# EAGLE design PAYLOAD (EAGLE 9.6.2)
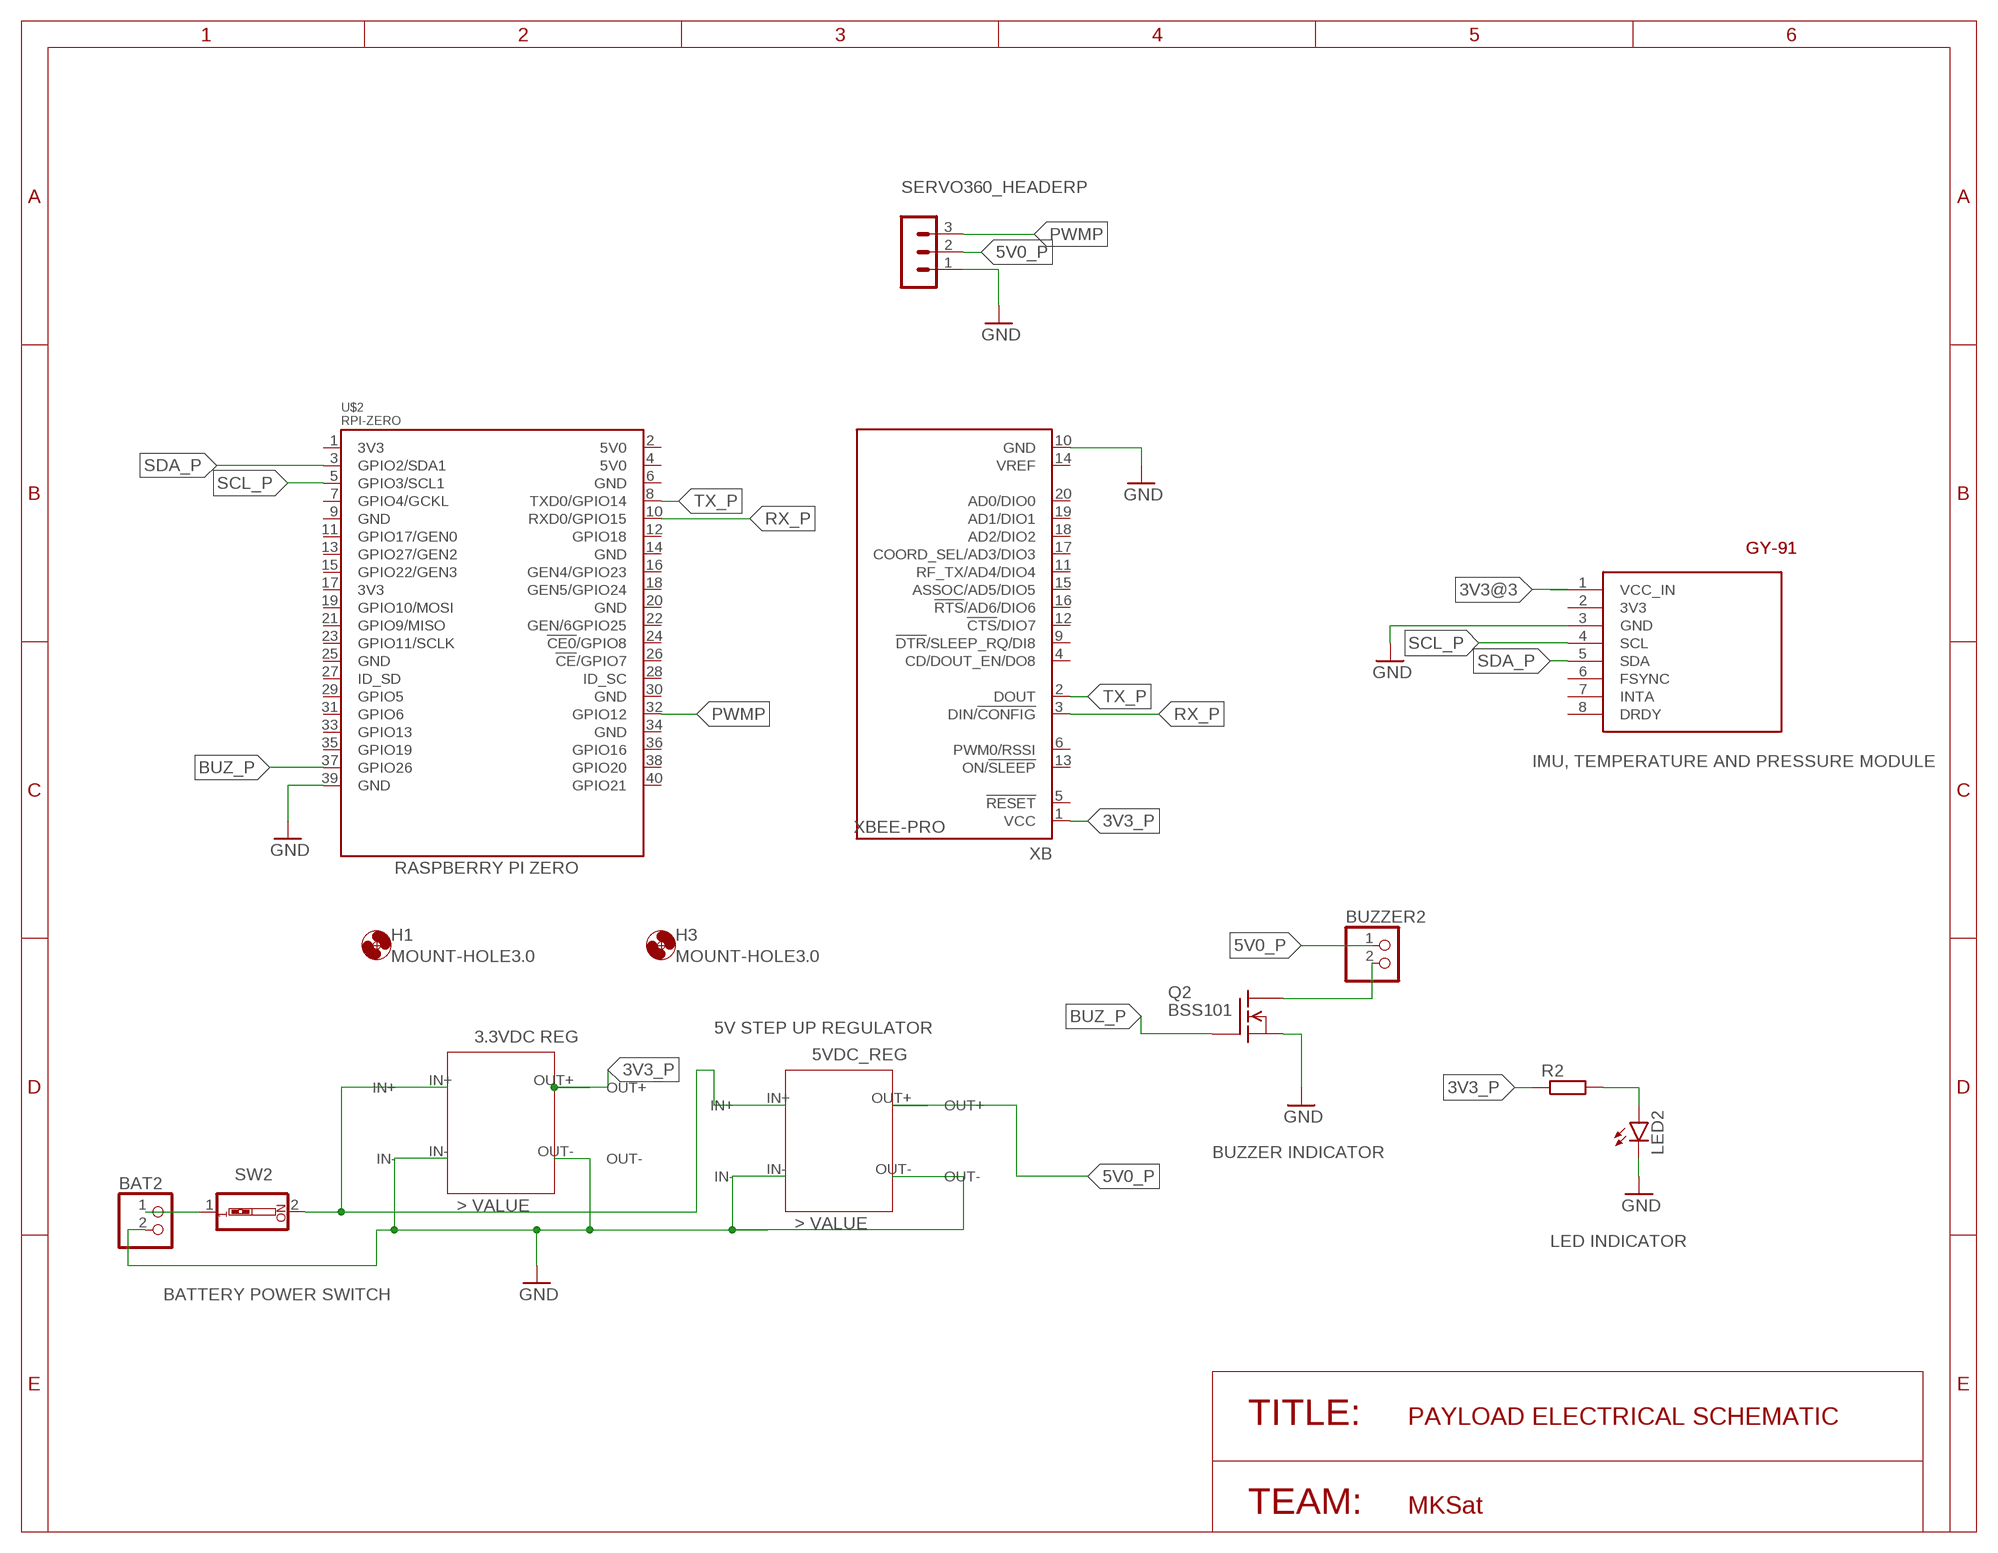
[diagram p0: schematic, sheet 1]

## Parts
BAT2  PINHD-1X2/90  [1X02/90]
BUZZER2  PINHD-1X2/90  [1X02/90]
GY-91  GY-86  [GY-86]
H1  MOUNT-HOLE3.0  [3,0]
H3  MOUNT-HOLE3.0  [3,0]
LED2  LED5MM  [LED5MM]
Q2  BSS101  [TO92]
R2  R-EU_0207/12  [0207/12]
SERVO360_HEADERP  MA03-1  [MA03-1]
SW2  SW_DIP-1  [EDG-01]
U$1  3VDC_REG  [3VDC_REG]
U$2  RPI-ZERO  [RASPBERRYPI_BASTELSTUBE_V13_RASPI_BOARD_B+_FULL]
U$3  5VDC_REG  [5VDC_REG]
XB  XBEE-PRO  [XBEE-PRO]

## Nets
3V3@3: GY-91.1(VCC_IN)
3V3_P: R2.1 U$1.OUT+ XB.1(VCC)
5V0_P: BUZZER2.1 SERVO360_HEADERP.2 U$3.OUT+
BUZ_P: Q2.2(G) U$2.37(GPIO26)
GND: BAT2.2 GY-91.3(GND) LED2.K(C) Q2.1(S) SERVO360_HEADERP.1 U$1.IN- U$1.OUT- U$2.39(GND) U$3.IN- U$3.OUT- XB.10(GND)
N$1: BUZZER2.2 Q2.3(D)
N$2: SW2.2 U$1.IN+ U$3.IN+
N$3: BAT2.1 SW2.1
N$11: LED2.A R2.2
PWMP: SERVO360_HEADERP.3 U$2.32(GPIO12)
RX_P: U$2.10(RXD0/GPIO15) XB.3(DIN/!CONFIG)
SCL_P: GY-91.4(SCL) U$2.5(GPIO3/SCL1)
SDA_P: GY-91.5(SDA) U$2.3(GPIO2/SDA1)
TX_P: U$2.8(TXD0/GPIO14) XB.2(DOUT)
Unconnected: GY-91.2(3V3) GY-91.6(FSYNC) GY-91.7(INTA) GY-91.8(DRDY) U$2.1(3V3) U$2.2(5V0) U$2.4(5V0) U$2.6(GND) U$2.7(GPIO4/GCKL) U$2.9(GND) U$2.11(GPIO17/GEN0) U$2.12(GPIO18) U$2.13(GPIO27/GEN2) U$2.14(GND) U$2.15(GPIO22/GEN3) U$2.16(GEN4/GPIO23) U$2.17(3V3) U$2.18(GEN5/GPIO24) U$2.19(GPIO10/MOSI) U$2.20(GND) U$2.21(GPIO9/MISO) U$2.22(GEN/6GPIO25) U$2.23(GPIO11/SCLK) U$2.24(!CE0!/GPIO8) U$2.25(GND) U$2.26(!CE!/GPIO7) U$2.27(ID_SD) U$2.28(ID_SC) U$2.29(GPIO5) U$2.30(GND) U$2.31(GPIO6) U$2.33(GPIO13) U$2.34(GND) U$2.35(GPIO19) U$2.36(GPIO16) U$2.38(GPIO20) U$2.40(GPIO21) XB.4(CD/DOUT_EN/DO8) XB.5(!RESET) XB.6(PWM0/RSSI) XB.9(!DTR!/SLEEP_RQ/DI8) XB.11(RF_TX/AD4/DIO4) XB.12(!CTS!/DIO7) XB.13(ON/!SLEEP) XB.14(VREF) XB.15(ASSOC/AD5/DIO5) XB.16(!RTS!/AD6/DIO6) XB.17(COORD_SEL/AD3/DIO3) XB.18(AD2/DIO2) XB.19(AD1/DIO1) XB.20(AD0/DIO0)

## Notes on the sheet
- GY-91 | GY-91
- IMU, TEMPERATURE AND PRESSURE MODULE
- RASPBERRY PI ZERO
- 5V STEP UP REGULATOR
- BUZZER INDICATOR
- LED INDICATOR
- BATTERY POWER SWITCH
- TITLE: | PAYLOAD ELECTRICAL SCHEMATIC
- TEAM: | MKSat

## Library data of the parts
BAT2 BUZZER2 = pinhead:PINHD-1X2: PIN HEADER
GY-91 = GY_Boards:GY-86
H1 H3 = holes:MOUNT-HOLE: MOUNTING HOLE with drill center marker
LED2 = led:LED: LED
Q2 = transistor-fet:BSS101: N-Channel Enhancement MOSFET 200V; 0,16A; 11Ohm
R2 = rcl:R-EU_: RESISTOR, European symbol; SPICEPREFIX: R
SERVO360_HEADERP = con-lstb:MA03-1: PIN HEADER; OC_FARNELL: unknown; OC_NEWARK: unknown
SW2 = special:SW_DIP-1: DIP SWITCH
U$1 = VOLTAGE_REGULATORS_CANSAT:3VDC_REG
U$2 = RPI-Zero:RPI-ZERO
U$3 = VOLTAGE_REGULATORS_CANSAT:5VDC_REG
XB = maxstream:XBEE: XBee (TM) /XBee-PRO(TM) OEM RF Modules Source: MaxStream, Inc. xbee_productmanual.pdf; MPN: XBP24-AWI-001; OC_FARNELL: 1337916; OC_NEWARK: 42M2667

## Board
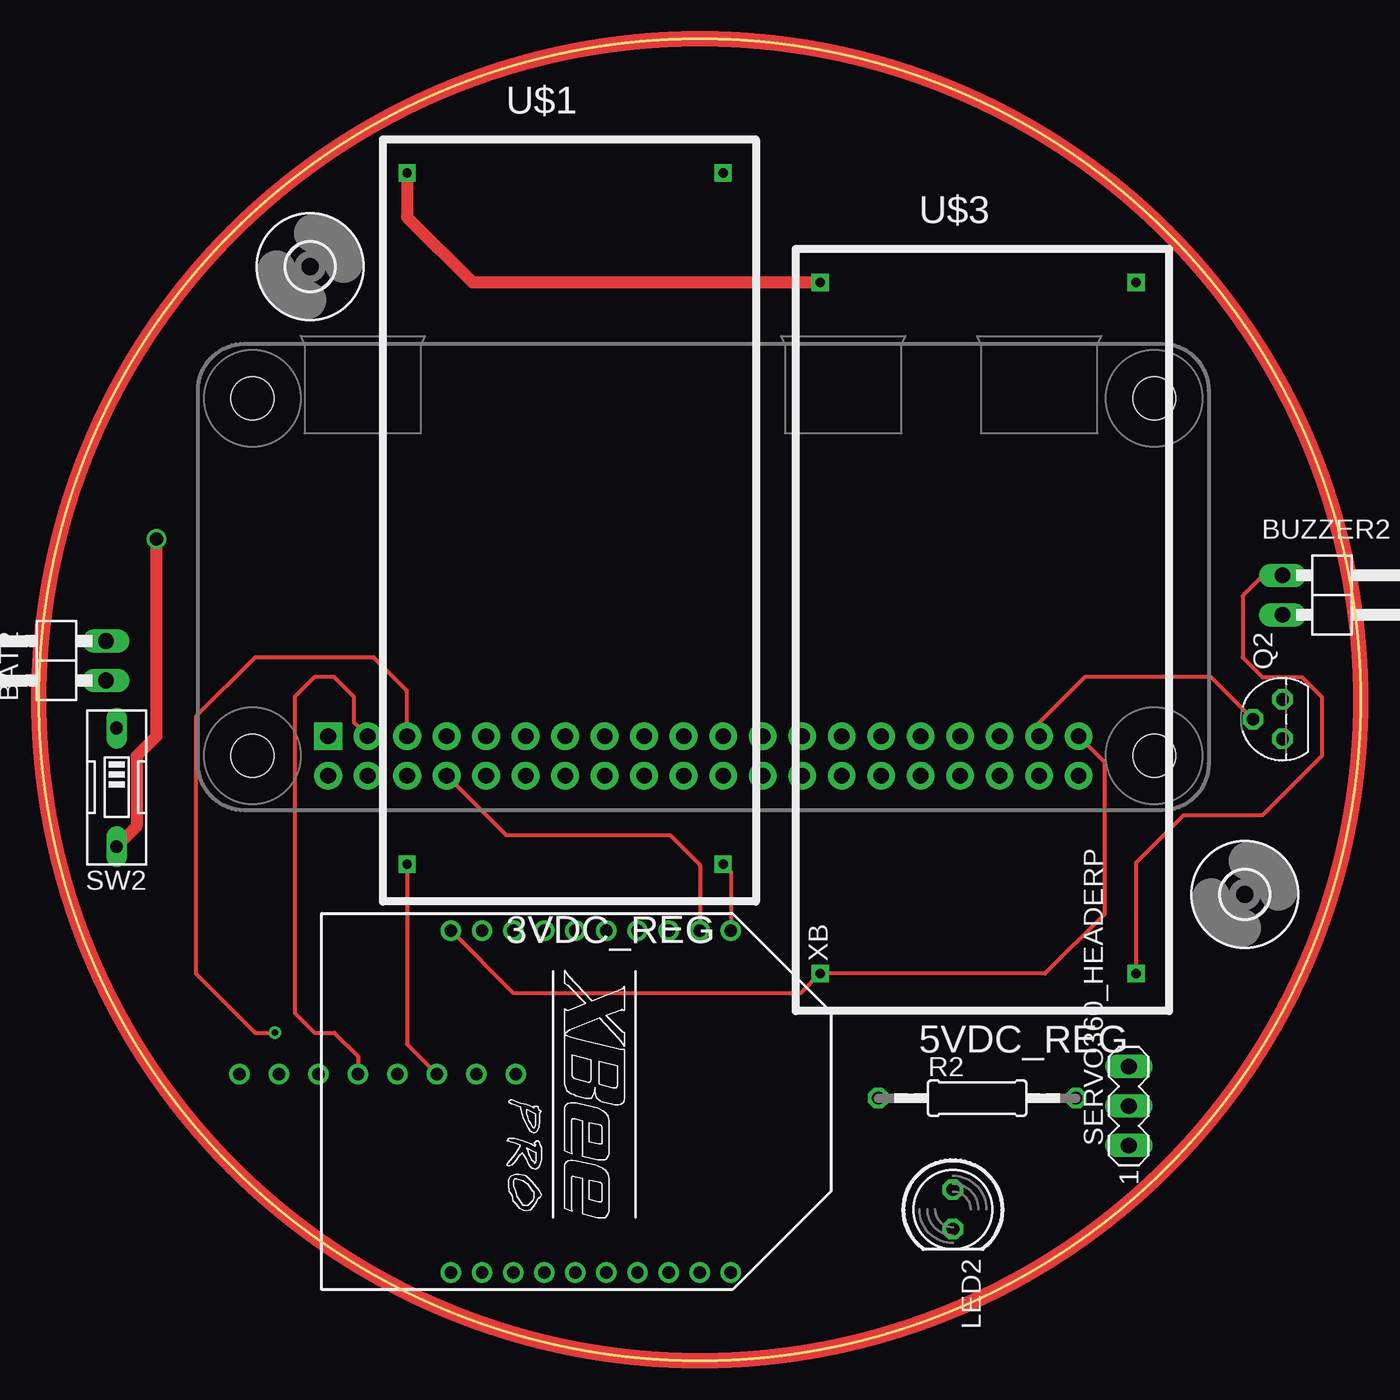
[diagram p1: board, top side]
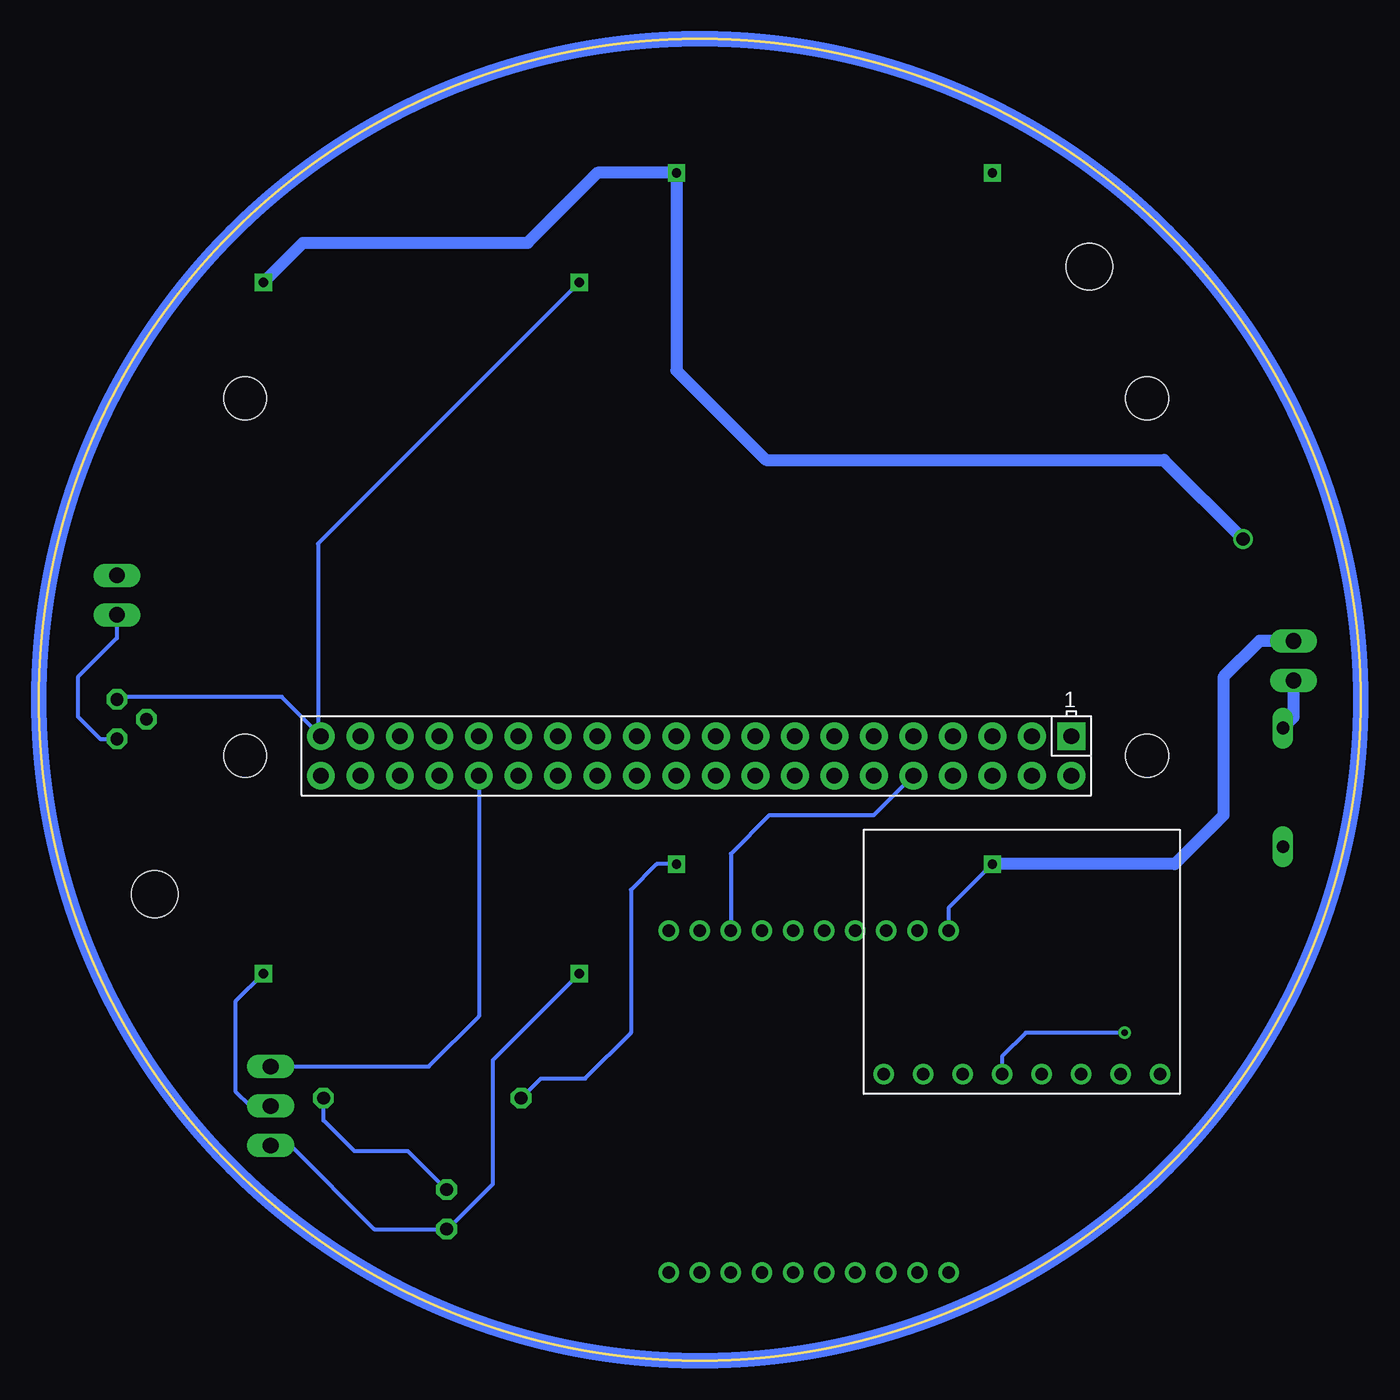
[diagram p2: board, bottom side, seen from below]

Size 85 x 85 mm. Coordinates in mm from the lower left corner, seen from the top.
Outline: circle at 42.5,42.5 radius 42.5
Copper layers (1*16): Top 0.035mm / dielectric 1.5mm / Bottom 0.035mm
Design rules "default *": minimum track width 6mil, minimum drill 0.35mm, track to track 12mil, track to pad 12mil, pad to pad 12mil, via to via 12mil, smd to smd 12mil, copper to edge 40mil, drill to drill 6mil, minimum pad ring 10mil, minimum via ring 8mil, stop-mask expansion 4mil, vias tented up to drill 0mil, thermal gap 10mil

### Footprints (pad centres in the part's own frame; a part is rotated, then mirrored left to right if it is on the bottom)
1X02/90 = drill 1.016 long: 1 -1.27,-3.81; 2 1.27,-3.81
GY-86 = drill 0.8: 1 1.27,19.05; 2 1.27,16.51; 3 1.27,13.97; 4 1.27,11.43; 5 1.27,8.89; 6 1.27,6.35; 7 1.27,3.81; 8 1.27,1.27
3,0 = hole 3: 0,0
LED5MM = drill 0.813 octagon: A -1.27,0; K 1.27,0
TO92 = drill 0.813 octagon: 1 1.27,0; 2 0,1.905; 3 -1.27,0
0207/12 = drill 0.813 octagon: 1 -6.35,0; 2 6.35,0
MA03-1 = drill 1.016 long: 1 -2.54,0; 2 0,0; 3 2.54,0
EDG-01 = drill 0.813 long: 1 0,-3.81; 2 0,3.81
3VDC_REG = drill 0.6 square: IN+ -22.86,8.89; IN- -22.86,-11.43; OUT+ 21.59,8.89; OUT- 21.59,-11.43
RASPBERRYPI_BASTELSTUBE_V13_RASPI_BOARD_B+_FULL = drill 1 pad 1.778 square: 1 8.37,25.23 | drill 1 pad 1.778: 2 8.37,27.77; 3 10.91,25.23; 4 10.91,27.77; 5 13.45,25.23; 6 13.45,27.77; 7 15.99,25.23; 8 15.99,27.77; 9 18.53,25.23; 10 18.53,27.77; 11 21.07,25.23; 12 21.07,27.77; 13 23.61,25.23; 14 23.61,27.77; 15 26.15,25.23; 16 26.15,27.77; 17 28.69,25.23; 18 28.69,27.77; 19 31.23,25.23; 20 31.23,27.77; 21 33.77,25.23; 22 33.77,27.77; 23 36.31,25.23; 24 36.31,27.77; 25 38.85,25.23; 26 38.85,27.77; 27 41.39,25.23; 28 41.39,27.77; 29 43.93,25.23; 30 43.93,27.77; 31 46.47,25.23; 32 46.47,27.77; 33 49.01,25.23; 34 49.01,27.77; 35 51.55,25.23; 36 51.55,27.77; 37 54.09,25.23; 38 54.09,27.77; 39 56.63,25.23; 40 56.63,27.77 | hole 2.75: 3.5,3.5; 3.5,26.5; 61.5,3.5; 61.5,26.5
5VDC_REG = drill 0.6 square: IN+ -22.86,8.89; IN- -22.86,-11.43; OUT+ 21.59,8.89; OUT- 21.59,-11.43
XBEE-PRO = drill 0.8 pad 1.27: 1 -11,9; 2 -11,7; 3 -11,5; 4 -11,3; 5 -11,1; 6 -11,-1; 7 -11,-3; 8 -11,-5; 9 -11,-7; 10 -11,-9; 11 11,-9; 12 11,-7; 13 11,-5; 14 11,-3; 15 11,-1; 16 11,1; 17 11,3; 18 11,5; 19 11,7; 20 11,9

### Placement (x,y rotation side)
BAT2  0.51,45.01 90 top
BUZZER2  83.79,49.23 270 top
GY-91  11.63,17.15 90 bottom
H1  17.44,70.36 0 top
H3  77.56,29.99 0 top
LED2  58.78,9.72 270 top
Q2  79.98,41.25 90 top
R2  60.34,16.88 0 top
SERVO360_HEADERP  70.09,16.37 90 top
SW2  5,36.87 180 top
U$1  35.11,53.52 270 top
U$2  10.23,65.39 180 bottom
U$3  61.67,46.48 270 top
XB  35.5,16.66 270 top

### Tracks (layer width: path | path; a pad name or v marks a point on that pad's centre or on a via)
3V3_P
  Top 0.254: U$1.OUT+ 44.5,31.43 XB.1
  Bottom 0.254: U$1.OUT+ 45.27,31.93 46.93,30.27 46.93,21.09 49.87,18.15 52.72,18.15 R2.1
5V0_P
  Top 0.254: BUZZER2.1 78.71,50.5 77.41,49.2 77.41,45.22 78.68,43.95 81.22,43.95 82.49,42.68 82.49,38.87 78.68,35.06 73.6,35.06 70.56,32.02 U$3.OUT+
  Bottom 0.254: SERVO360_HEADERP.2 71.42,16.37 72.33,17.28 72.33,23.12 U$3.OUT+
BUZ_P
  Top 0.254: Q2.2 75.38,43.95 67.25,43.95 64.32,41.02 U$2.37
GND
  Top 0.254: U$1.OUT- 23.68,20.34 GY-91.3 | U$2.39 68.52,38.5 68.52,28.71 64.7,24.89 U$3.OUT- 48.98,23.63 30.53,23.63 XB.10
  Top 0.762: U$1.IN- 23.68,73.55 27.89,69.34 U$3.IN-
  Bottom 0.254: SERVO360_HEADERP.1 68.82,13.83 63.44,8.45 LED2.K 58.78,8.39 55.82,11.35 55.82,19.31 U$3.OUT- | U$2.39 67.04,40.34 | 67.04,40.34 69.38,42.68 79.82,42.68 Q2.1 | U$3.IN- 67.04,52.53 67.04,40.34 | U$1.OUT- 26.5,29.11 XB.10
  Bottom 0.762: BAT2.2 6.5,46.28 8.83,43.95 8.83,35.06 11.96,31.93 U$1.OUT-
N$1
  Bottom 0.254: BUZZER2.2 79.98,46.46 82.49,43.95 82.49,41.41 81.06,39.98 Q2.3
N$2  (via drill 0.85)
  Top 0.762: v7.56,52.84 7.56,40.14 6.29,38.87 6.29,34.35 SW2.2
  Bottom 0.762: U$3.IN+ 68.01,71.89 53.57,71.89 49.08,76.38 U$1.IN+ 44,63.68 38.24,57.92 12.64,57.92 v7.56,52.84
N$3
  Bottom 0.762: BAT2.1 4.32,41.36 SW2.1
N$11
  Bottom 0.254: LED2.A 61.26,13.47 64.71,13.47 66.69,15.45 R2.2
PWMP
  Bottom 0.254: SERVO360_HEADERP.3 59.93,18.91 56.7,22.14 U$2.32
RX_P
  Bottom 0.254: U$2.10 31.32,35.06 38.04,35.06 40.5,32.6 XB.3
SCL_P  (via drill 0.4)
  Top 0.254: U$2.5 23.68,43.07 21.53,45.22 13.91,45.22 10.1,41.41 10.1,24.9 13.91,21.09 v15.18,21.09
  Bottom 0.254: v15.18,21.09 21.53,21.09 23.06,19.56 GY-91.4
SDA_P
  Top 0.254: U$2.3 20.26,41.04 20.26,42.68 18.99,43.95 17.72,43.95 16.45,42.68 16.45,22.36 17.72,21.09 18.99,21.09 20.52,19.56 GY-91.5
TX_P
  Top 0.254: U$2.8 30.05,33.79 40.58,33.79 42.5,31.87 XB.2
(copper drawn outside any net)
  shapes: Bottom circle x1, Top circle x1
